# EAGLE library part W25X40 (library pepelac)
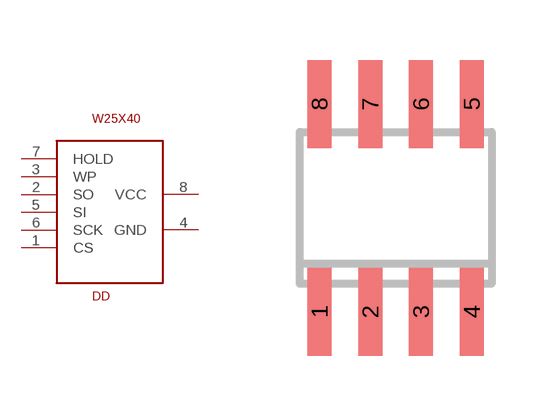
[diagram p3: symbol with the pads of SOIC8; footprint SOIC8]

Designator prefix DD

## W25X40  [SOIC8]
1  CS
2  SO
3  WP
4  GND
5  SI
6  SCK
7  HOLD
8  VCC

## Footprint SOIC8 (pad centres in mm)
Small Outline IC
smd 0.6 x 2.2: 1 -1.905,-2.6; 2 -0.635,-2.6; 3 0.635,-2.6; 4 1.905,-2.6; 5 1.905,2.6; 6 0.635,2.6; 7 -0.635,2.6; 8 -1.905,2.6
